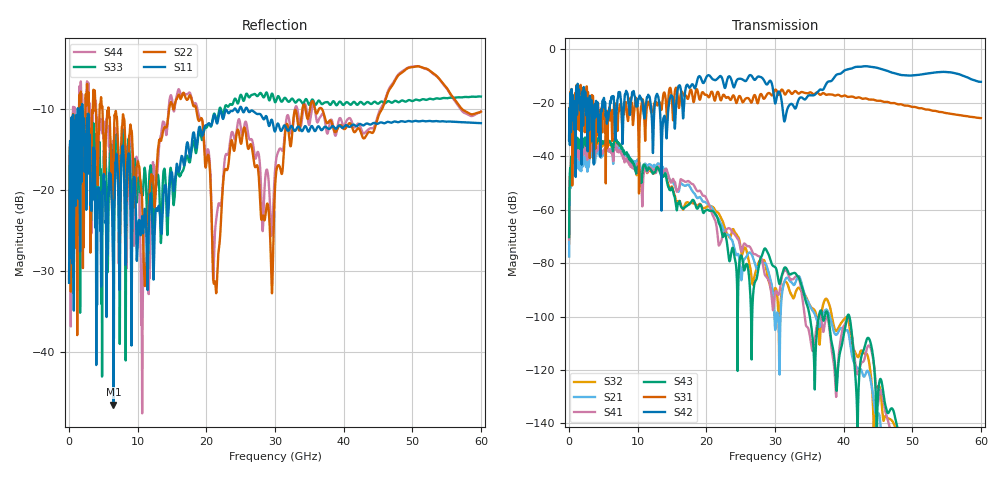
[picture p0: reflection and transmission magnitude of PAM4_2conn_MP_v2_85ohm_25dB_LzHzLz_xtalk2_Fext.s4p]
! Info: Touchstone file created by Circ.  Input file=FAB50GbE_2conn_Midplane_Examax_Topo2_v2_85ohm_25dB_LzHzLz.circ
# Hz S RI R 50
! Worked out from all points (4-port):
!   6000 points, 10 MHz to 60 GHz, reference 50 ohm
!   strongest paths, dB at 10 MHz, 15.01 GHz, 30.01 GHz, 45.01 GHz, 60 GHz:
!     S42: -34.0, -17.4, -20.2, -7.0, -12.1
!     S31: -33.8, -19.8, -15.1, -19.2, -25.7
!     S43: -70.3, -51.8, -81.5, -129.5, -174.1
!     S41: -71.2, -49.2, -91.5, -133.0, -182.4
!     S21: -77.5, -49.0, -104.5, -136.2, -182.8
!     S32: -72.7, -51.4, -89.4, -126.2, -167.9
!   lowest |S11| = -46.5 dB at 6.47 GHz (marker M1), VSWR 1.01, Z = 50.1 + j0.472 ohm
!   |S11| at or under -10 dB: start of sweep to 1.265 GHz; 1.953 GHz to 24.02 GHz (22.06 GHz wide, 170 % of centre); 26 GHz to end of sweep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
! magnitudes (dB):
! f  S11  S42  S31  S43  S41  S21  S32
! 10 MHz  -31.4  -34.0  -33.8  -70.3  -71.2  -77.5  -72.7
! 1 GHz  -11.8  -21.8  -16.5  -33.5  -36.5  -39.9  -35.4
! 6.47 GHz  -46.5  -17.6  -23.0  -36.3  -41.6  -41.3  -37.5
! 10.63 GHz  -23.4  -19.0  -19.2  -47.9  -56.6  -50.3  -49.2
! 14.78 GHz  -18.1  -17.6  -14.5  -52.7  -49.5  -49.5  -52.4
! 24.52 GHz  -10.3  -11.2  -19.3  -94.6  -70.8  -76.8  -69.9
! 60 GHz  -11.7  -12.1  -25.7  -174.1  -182.4  -182.8  -167.9
